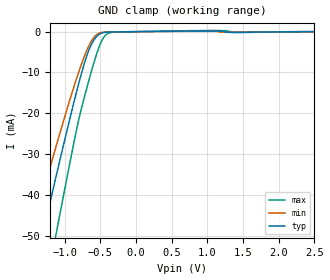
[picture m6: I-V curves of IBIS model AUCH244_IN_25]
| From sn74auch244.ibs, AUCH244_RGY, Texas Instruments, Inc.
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[Model]   AUCH244_IN_25
Model_type  Input
Vinl=0.7
Vinh=1.7
| variable   typ   min   max
C_comp   2.40pF   1.88pF   2.77pF
[Temperature Range]   40   100   -40
| Ambient temperature   25   85   -40
[Voltage range]   2.5   2.3   2.7
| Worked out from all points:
|   GND clamp passes 1 mA (typ) near -0.54 V on its own axis
[GND Clamp]
| AUCH244_IN_25
|   Voltage   I(typ)   I(min)   I(max)
-3.6V     -227.9mA   -191.3mA   -273.6mA
-1.455V   -61.08mA   -49.1mA    -80.31mA
-1.295V   -48.82mA   -39mA      -65.72mA
-1.105V   -34.47mA   -27.29mA   -48.4mA
-840mV    -15.31mA   -11.94mA   -24.73mA
-720mV    -7.65mA    -5.953mA   -15.89mA
-625mV    -3.191mA   -2.338mA   -9.815mA
-520mV    -732.2uA   -408.3uA   -3.951mA
-475mV    -336.9uA   -182.9uA   -2.115mA
-425mV    -161.1uA   -94.19uA   -847.9uA
-315mV    -73.99uA   -47.6uA    -145.2uA
2.5V      331.5pA    563.2nA    -12.81nA
